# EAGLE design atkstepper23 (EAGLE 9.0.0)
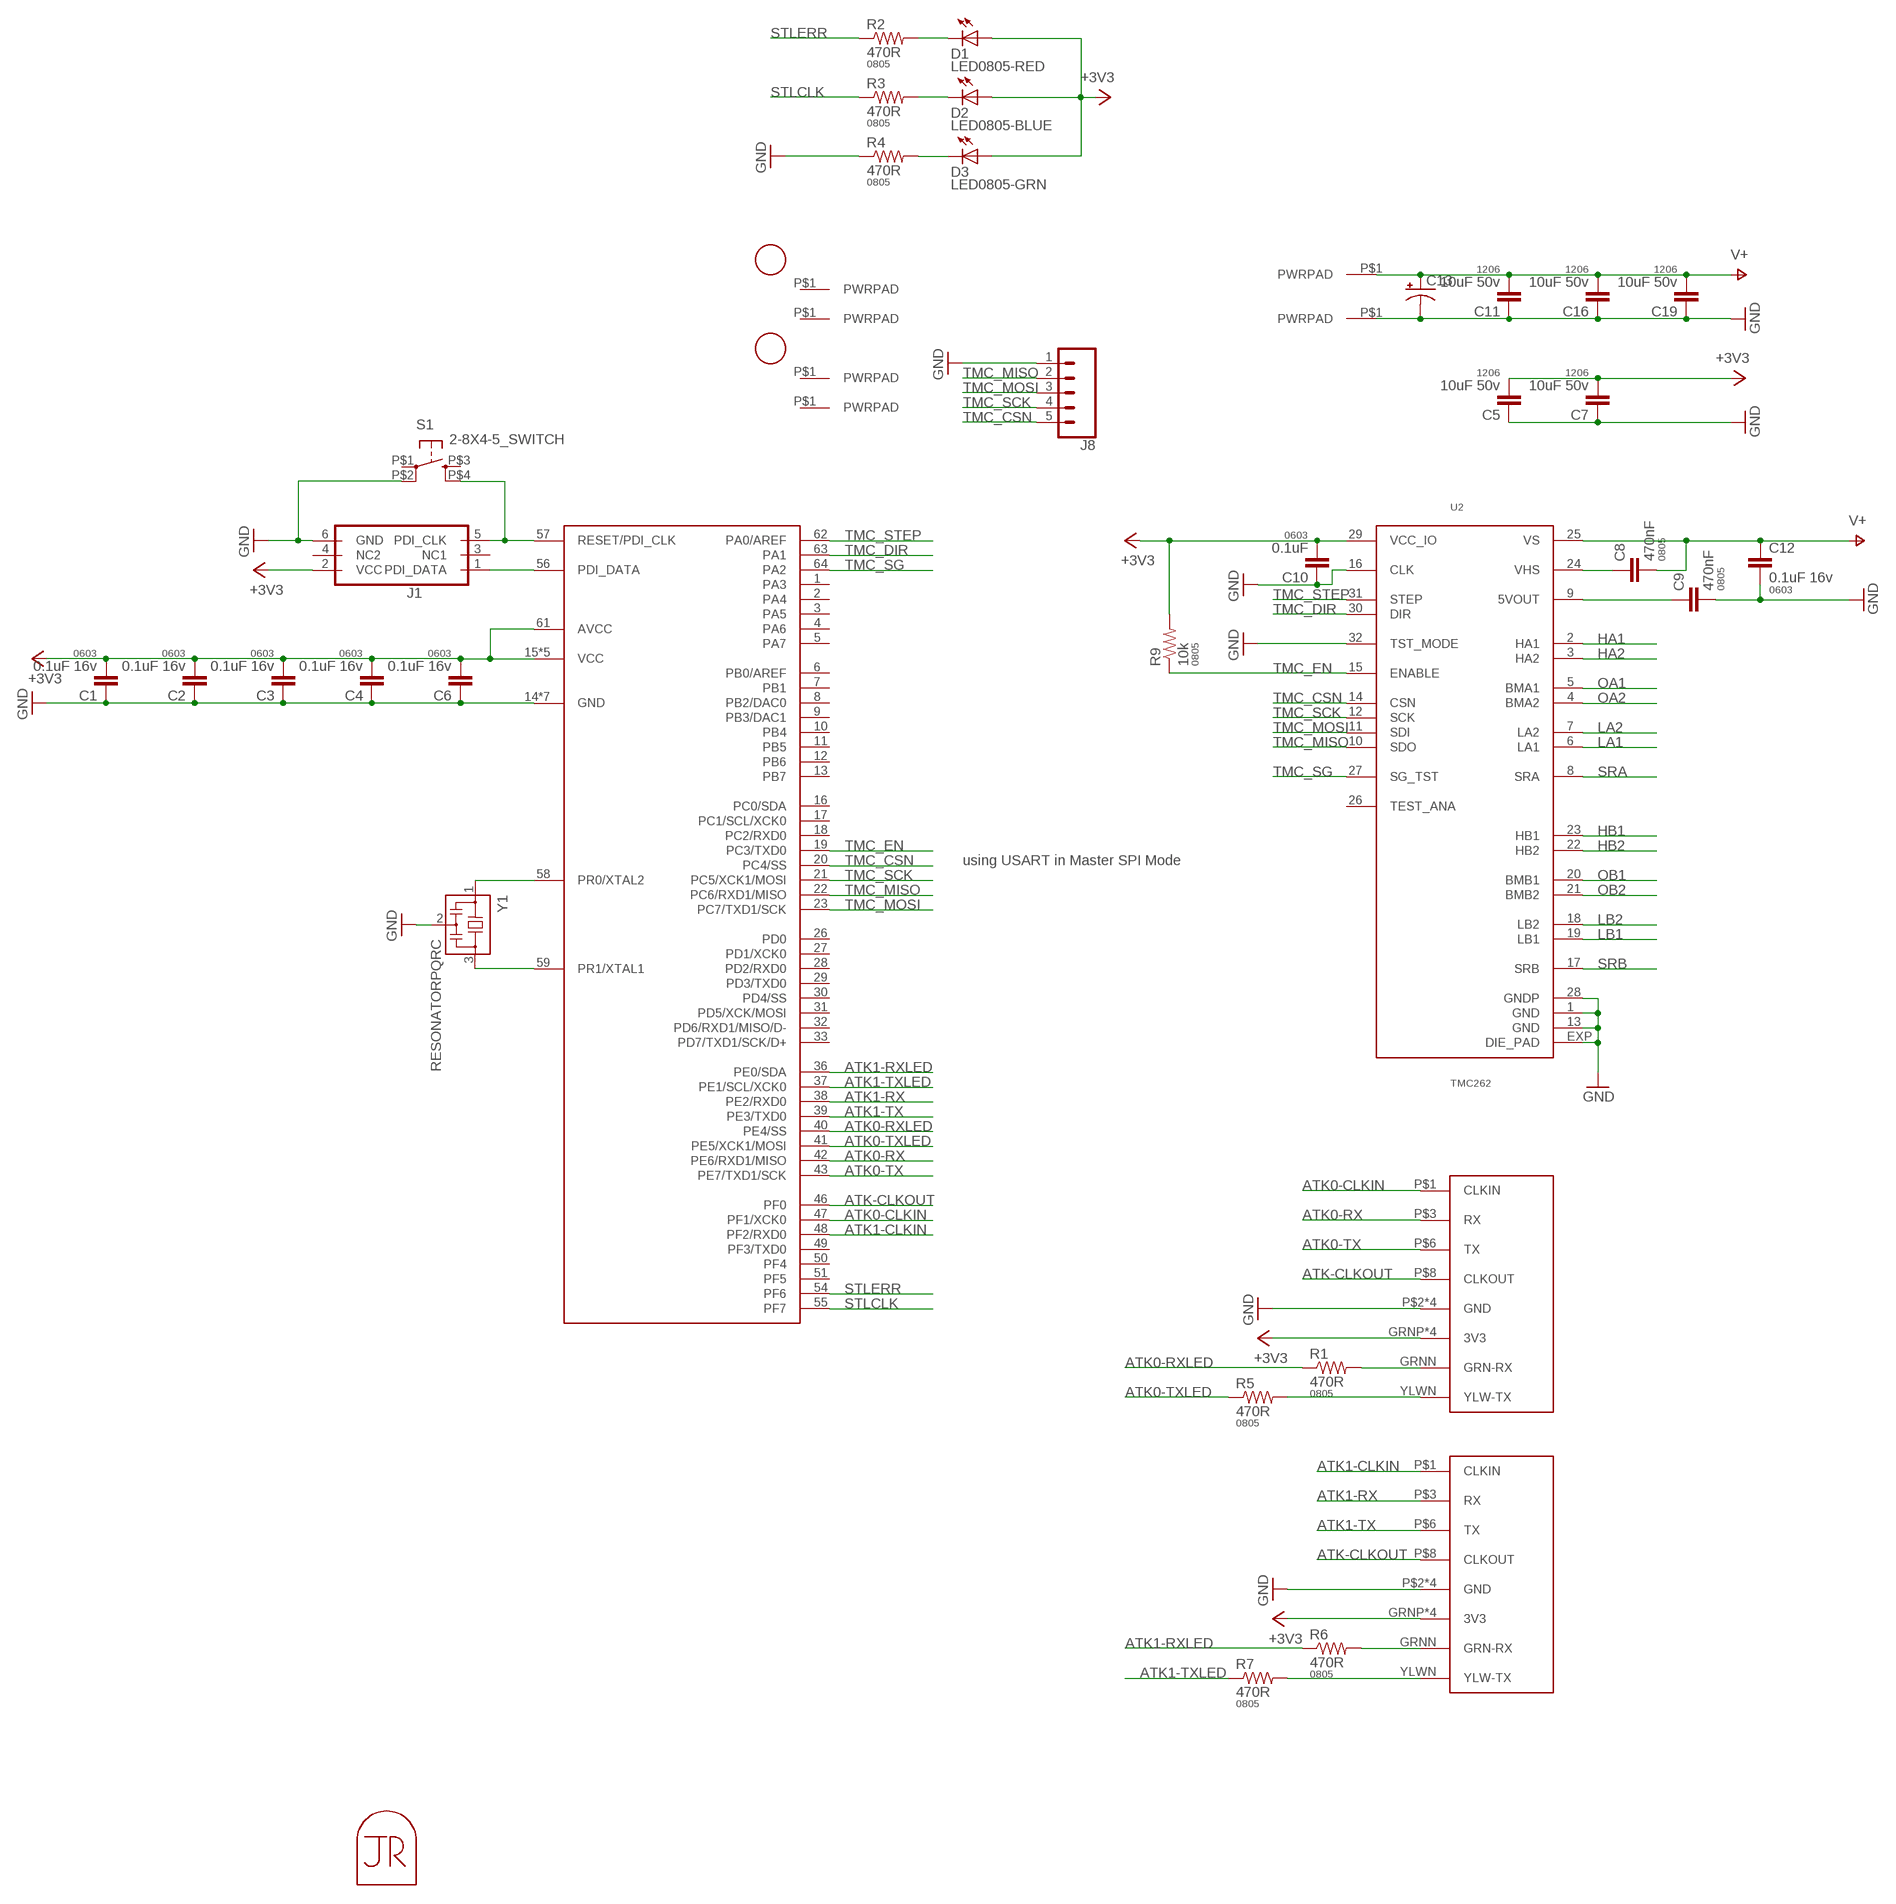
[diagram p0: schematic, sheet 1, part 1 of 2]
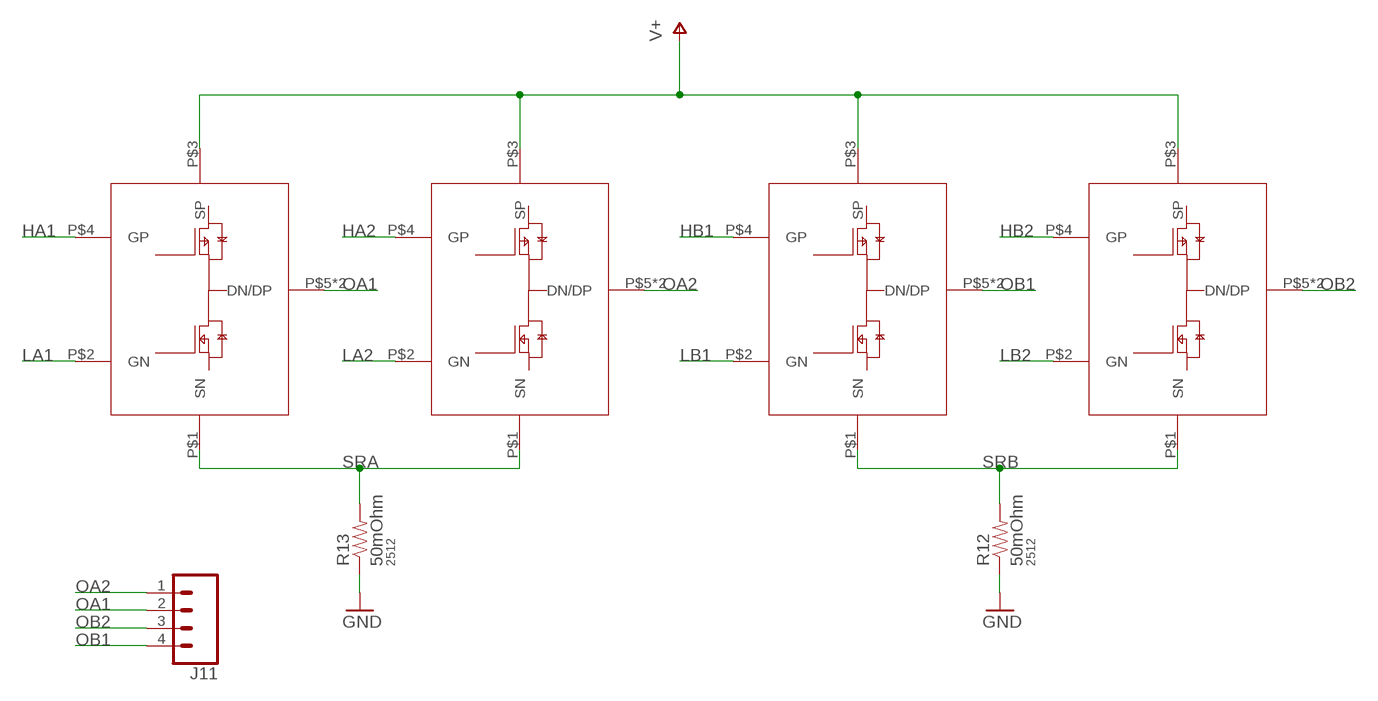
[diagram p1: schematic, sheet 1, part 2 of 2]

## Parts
C1  0.1uF 16v  CAP0603-CAP  [0603-CAP]
C2  0.1uF 16v  CAP0603-CAP  [0603-CAP]
C3  0.1uF 16v  CAP0603-CAP  [0603-CAP]
C4  0.1uF 16v  CAP0603-CAP  [0603-CAP]
C5  10uF 50v  CAP1206  [1206]
C6  0.1uF 16v  CAP0603-CAP  [0603-CAP]
C7  10uF 50v  CAP1206  [1206]
C8  470nF  CAP0805  [0805]
C9  470nF  CAP0805  [0805]
C10  0.1uF  CAP0603-CAP  [0603-CAP]
C11  10uF 50v  CAP1206  [1206]
C12  0.1uF 16v  CAP0603-CAP  [0603-CAP]
C13  CAP-POL-6.6X6.6  [6.6X6.6-CAP]
C16  10uF 50v  CAP1206  [1206]
C19  10uF 50v  CAP1206  [1206]
D1  LED0805-RED  LED0805  [LED0805]
D2  LED0805-BLUE  LED0805  [LED0805]
D3  LED0805-GRN  LED0805  [LED0805]
J1  PDIFEMALE_SMD  [PDI_2X3_SMD]
J2  ATK-PHY  [RJ45-LED-RJE7318800XXX]
J3  ATK-PHY  [RJ45-LED-RJE7318800XXX]
J4  PWRPADM3-SKINNY  [PWRPAD_3-25MM-SKINNY]
J6  PWRPADM3-SKINNY  [PWRPAD_3-25MM-SKINNY]
J8  CONN_05NO_SILK  [1X05_NO_SILK]
J9  PWRPAD  [PWRPAD_M3-PEM-MOUNT]
J10  PWRPAD  [PWRPAD_M3-PEM-MOUNT]
J11  CONN_04LONGPADS  [1X04_LONGPADS]
J12  PWRPADM3-SKINNY  [PWRPAD_3-25MM-SKINNY]
J13  PWRPADM3-SKINNY  [PWRPAD_3-25MM-SKINNY]
MP1  JRTOMBSTONE  [JRTOMBSTONE]
Q1  PNPAIR-STL40C30H3LL-FDD8424HSTM  [POWERFLAT-5X6]
Q2  PNPAIR-STL40C30H3LL-FDD8424HSTM  [POWERFLAT-5X6]
Q3  PNPAIR-STL40C30H3LL-FDD8424HSTM  [POWERFLAT-5X6]
Q4  PNPAIR-STL40C30H3LL-FDD8424HSTM  [POWERFLAT-5X6]
R1  470R  RESISTOR0805-RES  [0805]
R2  470R  RESISTOR0805-RES  [0805]
R3  470R  RESISTOR0805-RES  [0805]
R4  470R  RESISTOR0805-RES  [0805]
R5  470R  RESISTOR0805-RES  [0805]
R6  470R  RESISTOR0805-RES  [0805]
R7  470R  RESISTOR0805-RES  [0805]
R9  10k  RESISTOR0805-RES  [0805]
R12  50mOhm  RESISTOR2512  [R2512]
R13  50mOhm  RESISTOR2512  [R2512]
S1  2-8X4-5_SWITCH  [TACT-SWITCH-KMR6]
U1  ATXMEGA_A3UQFN  [QFN-64-9X9MM]
U2  TMC262  [QFN32]
U$1  FIDUCIAL  [FIDUCIAL_1MM]
U$2  FIDUCIAL  [FIDUCIAL_1MM]
Y1  RESONATORPQRC  [RES_PRQC]

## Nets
+3V3: C1.2 C2.2 C3.2 C4.2 C5.2 C6.2 C7.2 C10.2 D1.1(A) D2.1(A) D3.1(A) J1.2(VCC) J2.GRNP(3V3) J2.P$4(3V3) J2.P$5(3V3) J2.YLWP(3V3) J3.GRNP(3V3) J3.P$4(3V3) J3.P$5(3V3) J3.YLWP(3V3) R9.2 U1.15(VCC) U1.25(VCC) U1.35(VCC) U1.45(VCC) U1.53(VCC) U1.61(AVCC) U2.29(VCC_IO)
ATK0-CLKIN: J2.P$1(CLKIN) U1.47(PF1/XCK0)
ATK0-RX: J2.P$3(RX) U1.42(PE6/RXD1/MISO)
ATK0-RXLED: R1.1 U1.40(PE4/SS)
ATK0-TX: J2.P$6(TX) U1.43(PE7/TXD1/SCK)
ATK0-TXLED: R5.1 U1.41(PE5/XCK1/MOSI)
ATK1-CLKIN: J3.P$1(CLKIN) U1.48(PF2/RXD0)
ATK1-RX: J3.P$3(RX) U1.38(PE2/RXD0)
ATK1-RXLED: R6.1 U1.36(PE0/SDA)
ATK1-TX: J3.P$6(TX) U1.39(PE3/TXD0)
ATK1-TXLED: R7.1 U1.37(PE1/SCL/XCK0)
ATK-CLKOUT: J2.P$8(CLKOUT) J3.P$8(CLKOUT) U1.46(PF0)
GND: C1.1 C2.1 C3.1 C4.1 C5.1 C6.1 C7.1 C9.2 C10.1 C11.1 C12.2 C13.- C16.1 C19.1 J1.6(GND) J2.P$2(GND) J2.P$7(GND) J2.SHDL1(GND) J2.SHDL2(GND) J3.P$2(GND) J3.P$7(GND) J3.SHDL1(GND) J3.SHDL2(GND) J8.1 J10.P$1(PWRPAD) R4.1 R12.1 R13.1 S1.P$2(P1) U1.14(GND) U1.24(GND) U1.34(GND) U1.44(GND) U1.52(GND) U1.60(GND) U1.P$1(GND) U2.1(GND) U2.13(GND) U2.16(CLK) U2.28(GNDP) U2.32(TST_MODE) U2.EXP(DIE_PAD) Y1.2
HA1: Q1.P$4(GP) U2.2(HA1)
HA2: Q2.P$4(GP) U2.3(HA2)
HB1: Q3.P$4(GP) U2.23(HB1)
HB2: Q4.P$4(GP) U2.22(HB2)
LA1: Q1.P$2(GN) U2.6(LA1)
LA2: Q2.P$2(GN) U2.7(LA2)
LB1: Q3.P$2(GN) U2.19(LB1)
LB2: Q4.P$2(GN) U2.18(LB2)
N$1: D3.2(C) R4.2
N$2: C8.1 U2.24(VHS)
N$3: C9.1 U2.9(5VOUT)
N$4: J1.5(PDI_CLK) S1.P$4(S1) U1.57(RESET/PDI_CLK)
N$5: D2.2(C) R3.2
N$6: D1.2(C) R2.2
N$7: U1.58(PR0/XTAL2) Y1.1
N$8: U1.59(PR1/XTAL1) Y1.3
N$10: J1.1(PDI_DATA) U1.56(PDI_DATA)
N$11: J3.GRNN(GRN-RX) R6.2
N$12: J3.YLWN(YLW-TX) R7.2
N$17: J2.GRNN(GRN-RX) R1.2
N$18: J2.YLWN(YLW-TX) R5.2
OA1: J11.2 Q1.P$5(DN/DP) Q1.P$8(DN/DP) U2.5(BMA1)
OA2: J11.1 Q2.P$5(DN/DP) Q2.P$8(DN/DP) U2.4(BMA2)
OB1: J11.4 Q3.P$5(DN/DP) Q3.P$8(DN/DP) U2.20(BMB1)
OB2: J11.3 Q4.P$5(DN/DP) Q4.P$8(DN/DP) U2.21(BMB2)
SRA: Q1.P$1(SN) Q2.P$1(SN) R13.2 U2.8(SRA)
SRB: Q3.P$1(SN) Q4.P$1(SN) R12.2 U2.17(SRB)
STLCLK: R3.1 U1.55(PF7)
STLERR: R2.1 U1.54(PF6)
TMC_CSN: J8.5 U1.20(PC4/SS) U2.14(CSN)
TMC_DIR: U1.63(PA1) U2.30(DIR)
TMC_EN: R9.1 U1.19(PC3/TXD0) U2.15(ENABLE)
TMC_MISO: J8.2 U1.22(PC6/RXD1/MISO) U2.10(SDO)
TMC_MOSI: J8.3 U1.23(PC7/TXD1/SCK) U2.11(SDI)
TMC_SCK: J8.4 U1.21(PC5/XCK1/MOSI) U2.12(SCK)
TMC_SG: U1.64(PA2) U2.27(SG_TST)
TMC_STEP: U1.62(PA0/AREF) U2.31(STEP)
V+: C8.2 C11.2 C12.1 C13.+ C16.2 C19.2 J9.P$1(PWRPAD) Q1.P$3(SP) Q2.P$3(SP) Q3.P$3(SP) Q4.P$3(SP) U2.25(VS)
Unconnected: J1.3(NC1) J1.4(NC2) J4.P$1(PWRPAD) J6.P$1(PWRPAD) J12.P$1(PWRPAD) J13.P$1(PWRPAD) S1.P$1(P) S1.P$3(S) U1.1(PA3) U1.2(PA4) U1.3(PA5) U1.4(PA6) U1.5(PA7) U1.6(PB0/AREF) U1.7(PB1) U1.8(PB2/DAC0) U1.9(PB3/DAC1) U1.10(PB4) U1.11(PB5) U1.12(PB6) U1.13(PB7) U1.16(PC0/SDA) U1.17(PC1/SCL/XCK0) U1.18(PC2/RXD0) U1.26(PD0) U1.27(PD1/XCK0) U1.28(PD2/RXD0) U1.29(PD3/TXD0) U1.30(PD4/SS) U1.31(PD5/XCK/MOSI) U1.32(PD6/RXD1/MISO/D-) U1.33(PD7/TXD1/SCK/D+) U1.49(PF3/TXD0) U1.50(PF4) U1.51(PF5) U2.26(TEST_ANA)

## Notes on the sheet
- using USART in Master SPI Mode

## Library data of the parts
C1-C4 C6 C10 C12 = borkedlabs-passives:CAP: Capacitor; PACKAGE: 0603
C5 C7 C11 C16 C19 = borkedlabs-passives:CAP: Capacitor; PACKAGE: 1206
C8 C9 = borkedlabs-passives:CAP: Capacitor; PACKAGE: 0805
C13 = borkedlabs-passives:CAP-POL
D1-D3 = lights:LED: LED
J1 = microcontrollers:PDI: Multi connection point. Often used as Generic Header-pin footprint for 0.1 inch spaced/style header connections You can populate with any combo of single row headers, but if you'd like an exact match, check these: Header - 2x3 (Male, 0.1") (PRT-12807) Header - 2x3 (Female, 0.1") (PRT-13010) 2x3 Pin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; PROD_ID: CONN-11290
J2 J3 = connector:ATK-PHY
J4 J6 J9 J10 J12 J13 = power:PWRPAD
J8 = SparkFun-Connectors:CONN_05: Multi connection point. Often used as Generic Header-pin footprint for 0.1 inch spaced/style header connections On any of the 0.1 inch spaced packages, you can populate with these: Break Away Headers - Straight (PRT-00116) Break Away Male Headers - Right Angle (PRT-00553) Female Headers (PRT-00115)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
J11 = SparkFun-Connectors:CONN_04: Multi connection point. Often used as Generic Header-pin footprint for 0.1 inch spaced/style header connections On any of the 0.1 inch spaced packages, you can populate with these: Break Away Headers - Straight (PRT-00116) Break Away Male Headers - Right Angle (PRT-00553) Female Headers (PRT-00115)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; PROD_ID: CONN-09696
MP1 = connector:JRTOMBSTONE
Q1-Q4 = power:PNPAIR-STL40C30H3LL-FDD8424H
R1-R7 R9 = borkedlabs-passives:RESISTOR: Resistor; PACKAGE: 0805
R12 R13 = borkedlabs-passives:RESISTOR: Resistor; PACKAGE: 2512
S1 = fab:2-8X4-5_SWITCH
U1 = microcontrollers:ATXMEGA_A3U
U2 = power:TMC262
U$1 U$2 = connector:FIDUCIAL: For use by pick and place machines to calibrate the vision/machine, 1mm
Y1 = passives:RESONATOR

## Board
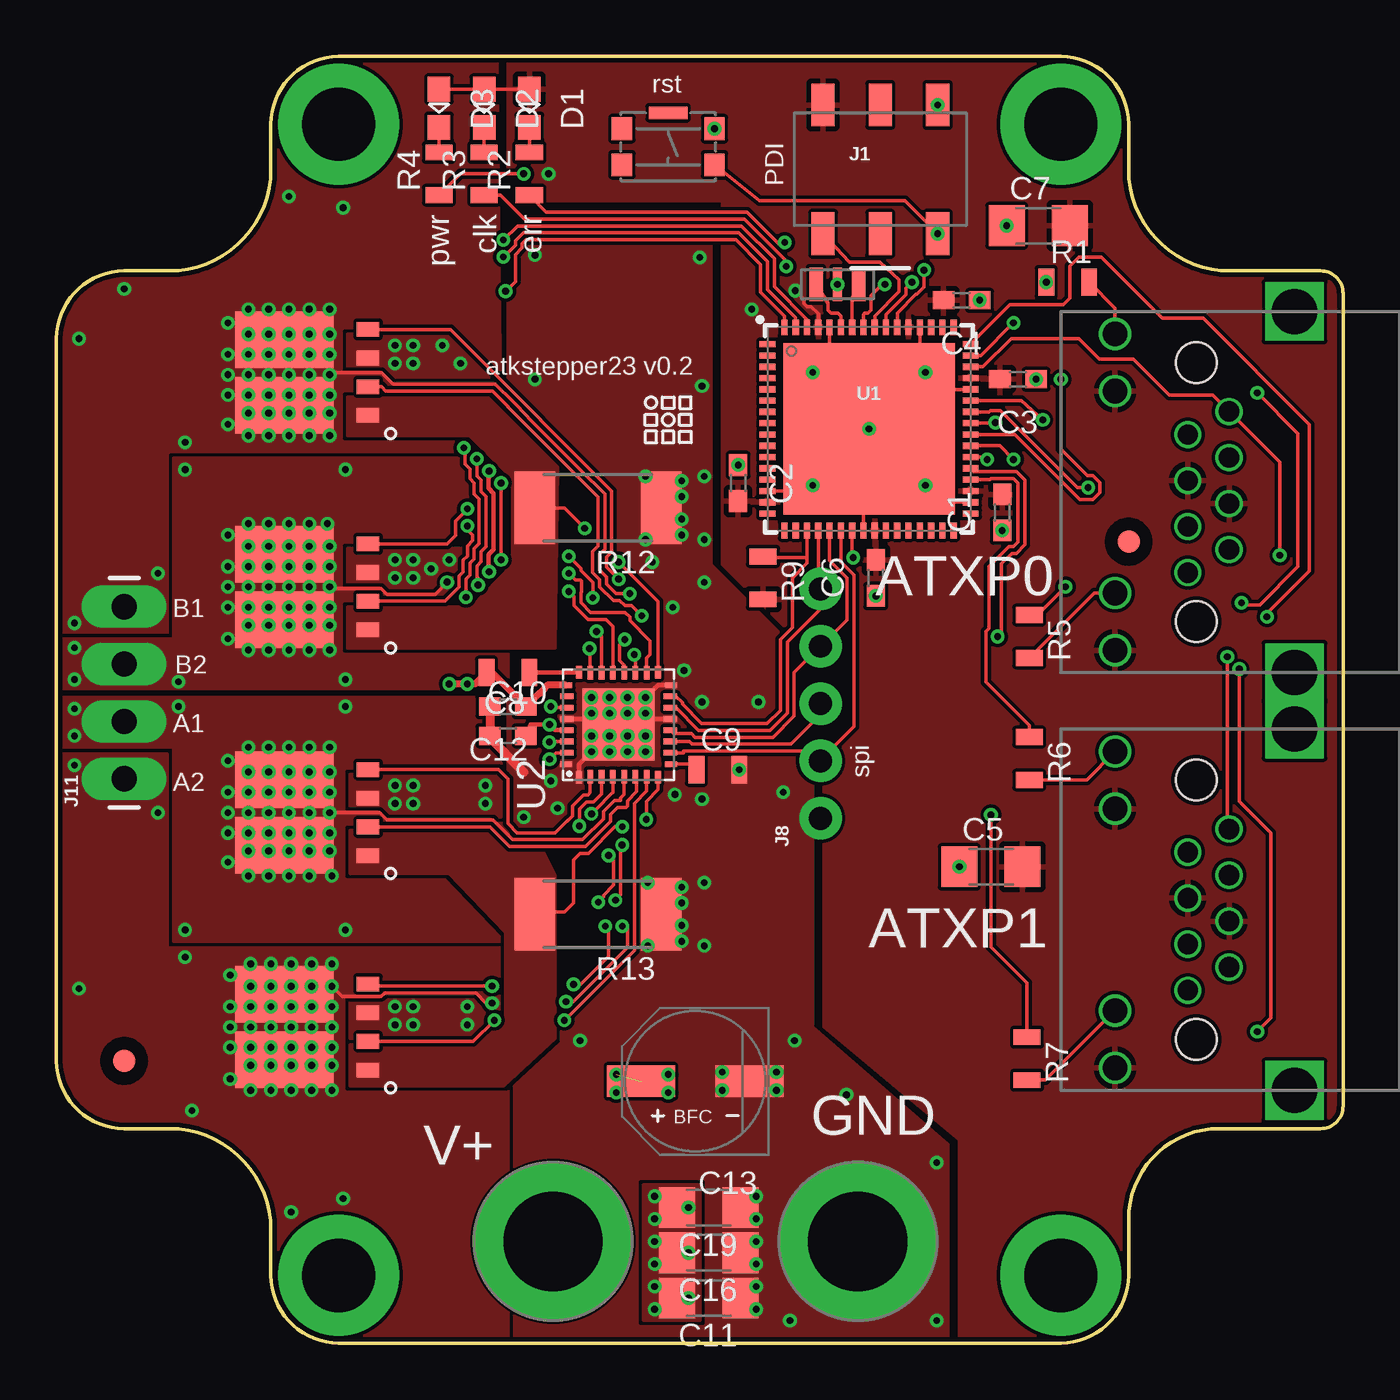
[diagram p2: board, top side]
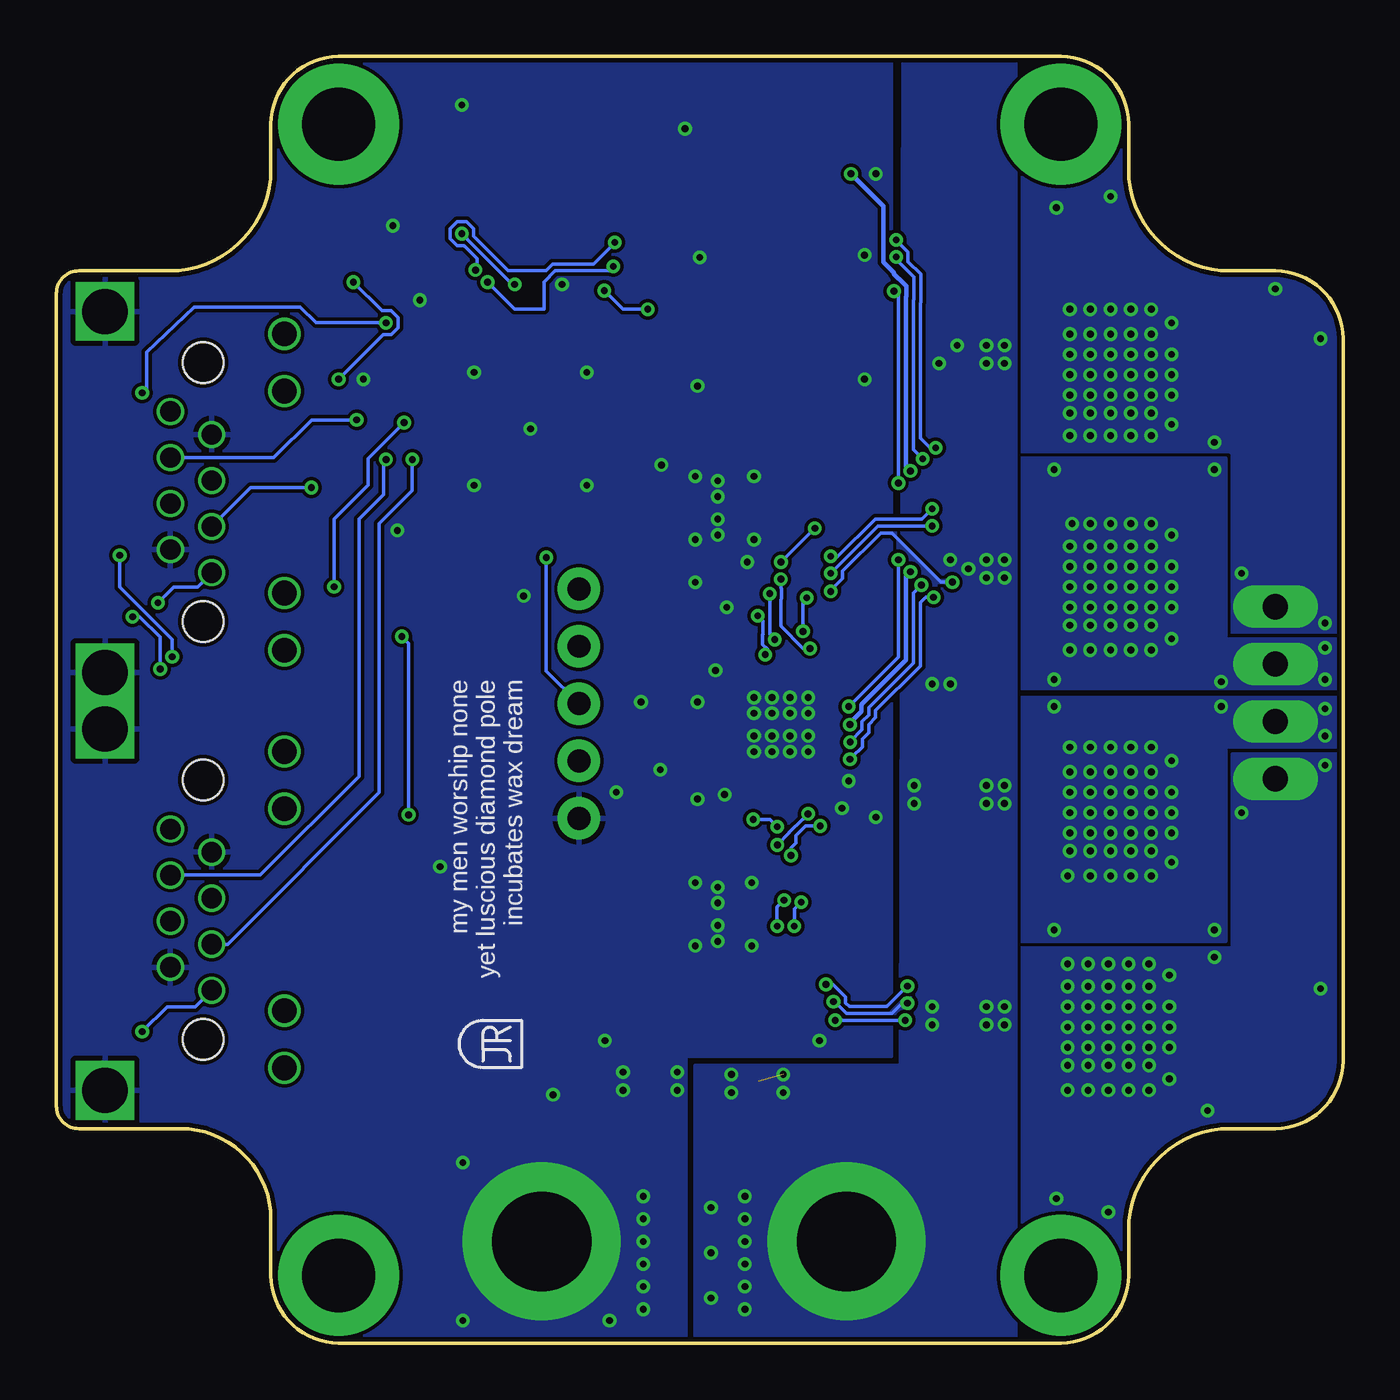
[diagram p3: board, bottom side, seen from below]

Size 57 x 57 mm. Coordinates in mm from the lower left corner, seen from the top.
Outline: 44.5,0 12.5,0 arc-90 9.5,3 9.5,5 arc90 5,9.5 3,9.5 arc-90 0,12.5 0,44.5 arc-90 3,47.5 5,47.5 arc90 9.5,52 9.5,54 arc-90 12.5,57 44.5,57 arc-90 47.5,54 47.5,52 arc90 52,47.5 56,47.5 arc-90 57,46.5 57,10.5 arc-90 56,9.5 51.5,9.5 arc90 47.5,5.5 47.5,3 arc-90 44.5,0
Copper layers (1*16): Top 0.035mm / dielectric 1.5mm / Bottom 0.035mm
Design rules "default *": minimum track width 6mil, minimum drill 0.3mm, track to track 6mil, track to pad 6mil, pad to pad 6mil, via to via 6mil, smd to smd 6mil, copper to edge 8mil, drill to drill 8mil, minimum pad ring 6mil, minimum via ring 6mil, stop-mask expansion 4mil, vias tented up to drill 27mil, thermal gap 9mil

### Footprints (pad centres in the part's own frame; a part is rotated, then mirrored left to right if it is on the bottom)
0603-CAP = smd 0.96 x 0.8: 1 -0.8,0; 2 0.8,0
1206 = smd 1.6 x 1.8: 1 -1.4,0; 2 1.4,0
0805 = smd 0.7 x 1.2: 1 -0.95,0; 2 0.95,0
6.6X6.6-CAP = smd 3 x 1.4: + 2.4,0; - -2.4,0
LED0805 = smd 1.1 x 1: 1 -0.85,0; 2 0.85,0
PDI_2X3_SMD = smd 1.02 x 1.9: 1 -2.54,-2.85; 2 -2.54,2.85; 3 0,-2.85; 4 0,2.85; 5 2.54,-2.85; 6 2.54,2.85
RJ45-LED-RJE7318800XXX = drill 1.1: GRNN 7.01,3.6; GRNP 4.47,3.6; YLWN -4.47,3.6; YLWP -7.01,3.6 | drill 0.9: P$1 -3.57,0.38; P$2 -2.55,-1.45; P$3 -1.53,0.38; P$4 -0.51,-1.45; P$5 0.51,0.38; P$6 1.53,-1.45; P$7 2.55,0.38; P$8 3.57,-1.45 | drill 2 square: SHDL1 -8,-4.35; SHDL2 8,-4.35 | hole 1.8: -5.74,0; 5.74,0
PWRPAD_3-25MM-SKINNY = drill 3.25 pad 5.35: P$1 0,0
1X05_NO_SILK = drill 1.016 pad 1.88: 1 0,0; 2 2.54,0; 3 5.08,0; 4 7.62,0; 5 10.16,0
PWRPAD_M3-PEM-MOUNT = drill 4.4 pad 7: P$1 0,0
1X04_LONGPADS = drill 1.118 pad 1.88 long: 1 0,0; 2 2.54,0; 3 5.08,0; 4 7.62,0
POWERFLAT-5X6 = smd 0.65 x 1: P$1 -1.905,-2.8; P$2 -0.635,-2.8; P$3 0.635,-2.8; P$4 1.905,-2.8 | smd 2.5 x 4.35: P$5 1.45,0.9; P$8 -1.45,0.9
R2512 = smd 1.8 x 3.2: 1 -2.8,0; 2 2.8,0
TACT-SWITCH-KMR6 = smd 0.9 x 1: P$1 -2.05,0.8; P$2 2.05,0.8; P$3 -2.05,-0.8; P$4 2.05,-0.8 | smd 1.7 x 0.55: P$5 0,1.5
QFN-64-9X9MM = smd 0.7 x 0.275: 1 -4.5,3.75; 2 -4.5,3.25; 3 -4.5,2.75; 4 -4.5,2.25; 5 -4.5,1.75; 6 -4.5,1.25; 7 -4.5,0.75; 8 -4.5,0.25; 9 -4.5,-0.25; 10 -4.5,-0.75; 11 -4.5,-1.25; 12 -4.5,-1.75; 13 -4.5,-2.25; 14 -4.5,-2.75; 15 -4.5,-3.25; 16 -4.5,-3.75; 33 4.5,-3.75; 34 4.5,-3.25; 35 4.5,-2.75; 36 4.5,-2.25; 37 4.5,-1.75; 38 4.5,-1.25; 39 4.5,-0.75; 40 4.5,-0.25; 41 4.5,0.25; 42 4.5,0.75; 43 4.5,1.25; 44 4.5,1.75; 45 4.5,2.25; 46 4.5,2.75; 47 4.5,3.25; 48 4.5,3.75 | smd 0.275 x 0.7: 17 -3.75,-4.5; 18 -3.25,-4.5; 19 -2.75,-4.5; 20 -2.25,-4.5; 21 -1.75,-4.5; 22 -1.25,-4.5; 23 -0.75,-4.5; 24 -0.25,-4.5; 25 0.25,-4.5; 26 0.75,-4.5; 27 1.25,-4.5; 28 1.75,-4.5; 29 2.25,-4.5; 30 2.75,-4.5; 31 3.25,-4.5; 32 3.75,-4.5; 49 3.75,4.5; 50 3.25,4.5; 51 2.75,4.5; 52 2.25,4.5; 53 1.75,4.5; 54 1.25,4.5; 55 0.75,4.5; 56 0.25,4.5; 57 -0.25,4.5; 58 -0.75,4.5; 59 -1.25,4.5; 60 -1.75,4.5; 61 -2.25,4.5; 62 -2.75,4.5; 63 -3.25,4.5; 64 -3.75,4.5 | smd 7.6 x 7.6: P$1 0,0
QFN32 = smd 0.55 x 0.25: 1 -2.325,1.75; 8 -2.325,-1.75; 17 2.325,-1.75; 24 2.325,1.75 | smd 0.6 x 0.25: 2 -2.3,1.25; 3 -2.3,0.75; 4 -2.3,0.25; 5 -2.3,-0.25; 6 -2.3,-0.75; 7 -2.3,-1.25; 18 2.3,-1.25; 19 2.3,-0.75; 20 2.3,-0.25; 21 2.3,0.25; 22 2.3,0.75; 23 2.3,1.25 | smd 0.25 x 0.55: 9 -1.75,-2.325; 16 1.75,-2.325; 25 1.75,2.325; 32 -1.75,2.325 | smd 0.25 x 0.6: 10 -1.25,-2.3; 11 -0.75,-2.3; 12 -0.25,-2.3; 13 0.25,-2.3; 14 0.75,-2.3; 15 1.25,-2.3; 26 1.25,2.3; 27 0.75,2.3; 28 0.25,2.3; 29 -0.25,2.3; 30 -0.75,2.3; 31 -1.25,2.3 | smd 3.2 x 3.2: EXP 0,0
FIDUCIAL_1MM = smd 1 x 1: 1 0,0
RES_PRQC = smd 0.6 x 1.5: 1 -0.95,0; 3 0.95,0 | smd 0.4 x 1.5: 2 0,0

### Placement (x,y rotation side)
C1  41.9,36.8 90 top
C2  30.2,38.1 270 top
C3  42.6,42.7 180 top
C4  40.1,46.2 180 top
C5  41.4,21.1 0 top
C6  36.3,33.9 90 top
C7  43.5,49.5 0 top
C8  20,29.7 180 top
C9  29.3,25.4 0 top
C10  20,26.9 0 top
C11  28.9,2 180 top
C12  20,28.2 180 top
C13  28.3,11.6 180 top
C16  28.9,4 180 top
C19  28.9,6 180 top
D1  20.95,54.7 270 top
D2  18.95,54.7 270 top
D3  16.95,54.7 270 top
J1  36.5,52 0 top
J2  50.5,37.7 90 top
J3  50.5,19.2 90 top
J4  12.5,3 180 top
J6  44.5,3 180 top
J8  33.85,23.25 90 top
J9  22,4.5 180 top
J10  35.5,4.5 180 top
J11  3,25 90 top
J12  12.5,54 180 top
J13  44.5,54 180 top
MP1  37.4,13.3 90 bottom
Q1  11,23.5 90 top
Q2  11,14 90 top
Q3  11,43 90 top
Q4  11,33.5 90 top
R1  44.8,47 0 top
R2  20.95,51.8 90 top
R3  18.95,51.8 90 top
R4  16.95,51.8 90 top
R5  43.1,31.3 270 top
R6  43.1,25.9 270 top
R7  43,12.6 270 top
R9  31.3,33.9 270 top
R12  24,37 180 top
R13  24,19 180 top
S1  27.1,53 0 top
U1  36,40.5 0 top
U2  24.9,27.4 90 top
U$1  3,12.5 0 top
U$2  47.5,35.5 0 top
U$5  [CBA-SILK-LOGO]  27.1,40.9 0 top
Y1  34.6,46.9 180 top

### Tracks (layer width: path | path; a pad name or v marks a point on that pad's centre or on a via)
+3V3  (via drill 0.3)
  Top 0.152: D1.1 D2.1 D3.1 | U1.61 33.75,45.6 33.43,45.92 33.26,45.92 33.12,46.05 33.12,46.23 v32.73,46.62
  Top 0.203: U2.29 22.09,27.15 v21.84,27.4 21,27.4 C10.2 | v19.16,34.16 19.16,34.45 19.14,34.47 19.14,34.93 19.37,35.16 19.37,37.64 19.14,37.87 19.14,38.33 19.16,38.35 v19.16,38.63
  Bottom 0.152: v32.73,46.62 31.9,45.8 v30.8,45.8
  Bottom 0.203: v21.84,27.4 21.84,27.47 21.34,27.97 21.34,28.29 19.37,30.26 19.37,33.96 v19.16,34.16 | v19.16,38.63 19.37,38.84 19.37,46.34 19.34,46.37 19.34,46.83 19.67,47.16 19.7,47.16 19.9,47.36 19.9,47.43 20.36,47.88 20.36,50.36 v21.8,51.8
  pour Top (rank 2): 20,58 20,50.6 29.5,50.6 29.5,34.5 34,30 34,14 40,9 40,-1 57.8,-0.8 57.8,58
ATK0-CLKIN  (via drill 0.3)
  Top 0.152: U1.47 40.95,43.75 v42.4,45.2 | v53.2,42.1 55,40.3 55,34.4 53.3,32.7 52.6,32.7 v52.5,32.8
  Bottom 0.152: v53.2,42.1 53,42.3 53,43.9 50.9,45.9 46.2,45.9 45.5,45.2 v42.4,45.2 | v52.5,32.8 51.8,33.5 50.75,33.5 J2.P$1
ATK0-RX  (via drill 0.3)
  Top 0.152: U1.42 41.32,41.25 41.38,41.31 41.82,41.31 45.23,37.9 v45.7,37.9
  Bottom 0.152: v45.7,37.9 48.39,37.9 J2.P$3
ATK0-RXLED  (via drill 0.3)
  Top 0.152: U1.40 42.45,40.25 45.33,37.37 45.92,37.37 46.23,37.68 46.23,38.12 45.92,38.43 45.68,38.43 44.5,39.61 v44.5,42.7
  Bottom 0.152: R1.1 42.58,45.73 42.18,45.73 41.87,45.42 41.87,44.98 42.18,44.67 42.53,44.67 v44.5,42.7
  other vias: 43.85,47
ATK0-TX  (via drill 0.3)
  Top 0.152: U1.43 42.75,41.75 v43.7,40.9
  Bottom 0.152: J2.P$6 47.37,39.23 45.7,40.9 v43.7,40.9
ATK0-TXLED  (via drill 0.3)
  Top 0.152: U1.41 41.57,40.75 v41.6,40.78 | v44.7,33.5 43.45,32.25 R5.1
  Bottom 0.152: v41.6,40.78 43.2,39.18 43.2,38 44.7,36.5 v44.7,33.5
ATK1-CLKIN  (via drill 0.3)
  Top 0.152: v53.2,13.8 53.8,14.4 53.8,22.6 52.4,24 v52.4,29.86 | U1.48 42.25,46 44.6,46 44.9,46.3 44.9,47.7 45.3,48.1 46.3,48.1 49,45.4 50.8,45.4 55.5,40.7 55.5,34.2 53.62,32.33 v53.62,32.17
  Bottom 0.152: v53.2,13.8 52.1,14.9 50.85,14.9 J3.P$1 | v53.62,32.17 53.31,32.17 52.4,31.27 v52.4,29.86
ATK1-RX  (via drill 0.3)
  Top 0.152: U1.38 41.13,39.25 v41.24,39.14
  Bottom 0.152: v41.24,39.14 41.24,37.76 42.7,36.3 42.7,24.39 49.42,17.67 J3.P$3
ATK1-RXLED
  Top 0.152: U1.36 41.35,38.25 41.41,38.31 42.4,38.31 42.6,38.1 42.6,35.5 42.4,35.29 42.19,35.29 41.3,34.4 41.3,31.65 41.17,31.52 41.17,29.28 43.1,27.35 R6.1
ATK1-TX  (via drill 0.3)
  Top 0.152: U1.39 41.79,39.75 v42.4,39.14
  Bottom 0.152: v42.4,39.14 42.5,39.04 42.5,37.6 43.6,36.5 43.6,25.1 47.97,20.73 J3.P$6
ATK1-TXLED  (via drill 0.3)
  Top 0.152: U1.37 40.63,38.62 40.95,38.62 40.95,38.61 42.52,38.61 42.91,38.23 42.91,35.37 42.52,34.99 42.32,34.99 41.87,34.53 41.87,31.47 v41.7,31.3 | v41.4,23.4 41.4,17.55 43,15.95 R7.1
  Bottom 0.152: v41.7,31.3 41.4,31 v41.4,23.4
ATK-CLKOUT  (via drill 0.3)
  Top 0.152: U1.46 41.05,43.25 42.3,44.5 45.3,44.5 46.2,43.6 47.7,43.6 49.3,42 51.22,42 J2.P$8 54.2,39.02 v54.2,34.9 | v51.87,30.4 51.87,23.19 J3.P$8
  Bottom 0.152: v54.2,34.9 54.2,33.5 51.87,31.17 v51.87,30.4
GND  (via drill 0.3)
  Top 0.152: R4.1 17.9,51.8 v20.7,51.8 | U1.60 34.25,42.25 35.9,40.6 | 35.9,40.6 U1.P$1 36.05,40.55 | U1.52 38.25,42.75 36.05,40.55 | U1.34 39.35,37.25 36.05,40.55 | U1.24 35.75,40.4 | 35.75,40.4 35.75,40.45 35.9,40.6 | U1.14 33.1,37.75 35.75,40.4 | U1.44 39.25,42.25 v38.5,43
  Top 0.203: U2.1 23.15,25.65 v23.7,26.2 | U2.13 26.35,27.65 v26.1,27.9 | U2.16 26.65,29.15 v26.1,28.6 | U2.28 23.45,27.65 v23.7,27.9
  Top 0.406: C12.2 C10.1 19.2,26.8 20.7,25.3
  other vias: 26.1,26.2 24.5,26.2 25.3,26.2 26.1,26.9 23.7,26.9 24.5,26.9 25.3,26.9 24.5,27.9 25.3,27.9 23.7,28.6 24.5,28.6 25.3,28.6 27.7,17.8 27.7,18.5 27.7,19.5 27.7,20.2 28.7,20.4 28.7,17.6 26.2,17.6 26.2,20.4 27.7,35.8 27.7,36.5 27.7,37.5 27.7,38.2 28.7,38.4 28.7,35.6 26.1,35.6 26.1,38.4 30.25,25.4 27.8,29.8 28.6,28.4 26.4,34.6 21.2,42.7 28.6,42.4 28.5,48.1 21.2,48.2 27.4,24.3 28.6,24.1 31.9,11.2 35,11 31.9,12 39,8 39,1 32.5,1 29.5,11.2 23.2,13.4 20.7,23.3 21.9,24.9 40.9,46.2 41.9,36 30.2,38.9 36.3,33.1 31,1.5 31,2.5 31,3.5 31,4.5 31,5.5 31,6.5 29.5,12 22.2,23.7 27.3,32.6 28.7,33.7 34.6,46.9 29.15,53.8 39.04,54.85 36,40.5 33.5,43 38.5,38 33.5,38 43.4,42.7 42.1,49.5 40,21.1 31.1,28.4 32.2,24.4 32.7,13.4
  pour Bottom: 29.1,-0.5 29.1,12.7 20,12.7 20,59.6 29.5,59.5 59.5,59.5 59,-0.5
  pour Top (no thermals): 25.8,35.3 29,35.3 29,38.7 25.8,38.7
  pour Top (no thermals): 25.8,17.3 29,17.3 29,20.7 25.8,20.7
  pour Top (rank 6, no thermals): 39.5,-1 39.5,8.8 33.5,14 33.5,30 29,34.5 29,50.1 20,50.1 20,-1
HA1
  Top 0.152: U2.2 23.65,24.39 23.54,24.28 23.36,24.28 22.86,23.79 22.86,23.36 22.64,23.13 22.64,23.14 22.1,22.61 20.4,22.61 20,23.01 20,25 19.59,25.41 Q1.P$4
HA2  (via drill 0.3)
  Top 0.152: v22.91,15.89 23.23,15.89 24.47,17.13 24.47,18.31 v24.31,18.47 | v24.01,19.53 24.23,19.76 24.23,19.84 24.69,20.29 24.69,21.37 v24.46,21.6 | v23.17,22.91 23.17,23.66 23.48,23.98 23.8,23.98 24.15,24.32 U2.3 | v19.3,15.81 13.89,15.81 Q2.P$4
  Bottom 0.152: v19.3,15.81 20.2,14.91 21.87,14.91 22.04,15.08 22.04,15.35 22.59,15.89 v22.91,15.89 | v24.31,18.47 24.31,19.23 v24.01,19.53 | v24.46,21.6 24.46,21.94 24.23,22.16 24.23,22.48 23.81,22.91 v23.17,22.91
HB1  (via drill 0.3)
  Top 0.152: v24.91,33.84 24.37,34.38 24.37,34.82 24.6,35.05 | 24.6,35.05 | 24.6,35.05 24.6,37.74 21.45,40.89 21.45,40.92 20.54,41.83 20.44,41.92 20.44,41.93 20.38,41.98 17.46,44.91 Q3.P$4 | U2.23 23.65,30.74 v23.62,30.77
  Bottom 0.152: v24.91,33.84 24.91,33.46 24.87,33.42 24.87,32.98 24.91,32.94 24.91,31.75 23.92,30.77 v23.62,30.77
HB2  (via drill 0.3)
  Top 0.152: v18.2,36.96 v18.2,36.95 17.67,36.42 17.67,35.77 17.3,35.4 Q4.P$4 | v22.7,34.86 v22.7,34.85 23.23,34.32 23.23,34.23 23.76,33.69 v23.76,33.02 | v23.93,31.53 24.15,31.31 U2.22
  Bottom 0.152: v18.2,36.96 18.66,36.51 20.73,36.51 22.42,34.82 22.66,34.82 v22.7,34.86 | v23.93,31.53 23.93,32.85 v23.76,33.02
LA1
  Top 0.152: U2.6 25.7,25.05 25.7,24.43 25.3,24.03 25.3,23.8 25.23,23.73 24.85,23.73 24.54,23.42 24.54,23.1 23.44,22 20.07,22 19.21,22.86 Q1.P$2
LA2  (via drill 0.3)
  Top 0.152: v22.5,14.3 25.6,17.4 25.6,23.9 26.15,24.45 U2.7 | Q2.P$2 18.46,13.37 v19.4,14.3
  Bottom 0.152: v19.4,14.3 v22.5,14.3
LB1  (via drill 0.3)
  Top 0.152: U2.19 25.65,30.45 v25.6,30.5 | v25.93,32.22 25.48,32.67 25.18,32.67 24.95,32.9 24.67,32.9 24.07,33.5 24.07,33.82 23.76,34.13 23.76,35.07 23.99,35.3 23.99,37.48 20.01,41.46 20.01,41.49 19.32,42.18 14.59,42.18 14.4,42.37 Q3.P$2
  Bottom 0.152: v25.6,30.5 25.5,30.6 25.5,30.74 25.71,30.95 25.71,31.39 25.7,31.4 25.7,31.99 v25.93,32.22
LB2  (via drill 0.3)
  Top 0.152: v18.2,36.2 18.2,36.03 18.43,35.8 18.43,35.55 18.2,35.32 18.2,34.87 18.02,34.69 18.02,34.16 17.84,33.97 17.84,33.49 17.21,32.87 Q4.P$2 | U2.18 26.15,30.35 26.3,30.5 26.3,31.1 25.4,32 25.4,32.16 25.2,32.36 23.67,32.36 23.23,32.8 23.23,33.24 23.26,33.27 23.26,33.76 23.23,33.8 23,33.8 v22.7,34.1
  Bottom 0.152: v18.2,36.2 20.6,36.2 v22.7,34.1
N$1
  Top 0.152: D3.2 R4.2
N$2
  Top 0.203: U2.24 23.12,29.7 C8.1
N$3
  Top 0.152: U2.9 28.35,25.65 C9.1
N$4  (via drill 0.3)
  Top 0.152: U1.57 35.75,45.57 35.8,45.62 35.95,45.62 36.08,45.76 36.08,46.4 36.58,46.9 v36.7,46.9 | S1.P$4 31.15,50.6 37.59,50.6 J1.5
  Bottom 0.152: J1.5 38.81,48.92 38.81,48.91 36.8,46.9 v36.7,46.9
  other vias: 39.04,49.15
N$5
  Top 0.152: D2.2 R3.2
N$6
  Top 0.152: D1.2 R2.2
N$7
  Top 0.152: U1.58 35.25,46.3 Y1.1
N$8
  Top 0.152: U1.59 34.75,45.5 34.63,45.62 34.3,45.62 34.17,45.76 34.17,46.08 Y1.3
N$10
  Top 0.152: J1.1 35.13,47.88 36.47,47.88 37.33,47.12 37.33,46.58 36.25,45.5 U1.56
N$11
  Top 0.152: J3.GRNN 45.64,24.95 R6.2
N$12
  Top 0.152: R7.2 43.82,11.65 J3.YLWN
N$17
  Top 0.152: R1.2 46.9,45.85 J2.GRNN
N$18
  Top 0.152: R5.2 45.98,33.23 J2.YLWN
OA1  (via drill 0.3)
  Top 0.152: U2.5 25.15,24.31 24.99,24.15 24.99,24.04 24.72,24.04 24.23,23.55 24.23,23.23 23.31,22.3 20.2,22.3 19.34,23.17 14.64,23.17 14.31,23.5 v12.1,23.5 | 10.51,22.99 Q1.P$5
  other vias: 7.6,21.3 7.6,22.6 7.6,23.5 7.6,24.4 7.6,25.8 12.1,21.8 12.2,20.7 12.1,26.4 12.1,25.3 11.2,21.8 11.2,22.6 11.2,23.5 11.2,24.4 11.2,25.3 10.3,21.8 10.3,20.7 10.3,23.5 10.3,26.4 10.3,25.3 9.4,21.8 9.4,22.6 9.4,23.5 9.4,24.4 9.4,25.3 8.5,21.8 8.5,20.7 8.5,23.5 8.5,26.4 8.5,25.3 12.8,28.2 5.4,28.2 0.8,28.1 0.8,26.9 5.7,18.3 12.8,18.3 8.5,22.6 10.3,22.6 12.1,22.6 11.2,20.7 9.4,20.7 10.3,24.4 12.1,24.4 8.5,24.4 9.4,26.4 11.2,26.4
  pour Top (rank 2, no thermals): -0.3,28.6 20,28.6 20,17.8 5.2,17.8 5.2,26.4 -0.3,26.4
  pour Bottom (rank 2, no thermals): -0.3,28.6 20,28.6 20,17.8 5.2,17.8 5.2,26.4 -0.3,26.4
OA2  (via drill 0.3)
  Top 0.152: v22.57,15.12 22.89,15.12 25.3,17.53 25.3,18.4 25.23,18.47 v25.07,18.47 | v24.76,19.62 24.99,19.85 24.99,22 v25.06,22.07 | U2.4 24.65,24.39 24.6,24.34 | 24.6,24.34 | 23.93,23.67 | 23.93,23.67 v23.7,23.45 | 24.6,24.34 23.93,23.67 | v19.3,15.06 19.04,15.06 18.59,15.51 14.55,15.51 14.39,15.35 12.65,15.35 v12.2,15.8
  Bottom 0.152: v19.3,15.06 19.54,15.06 20,14.61 22,14.61 22.52,15.12 v22.57,15.12 | v25.07,18.47 25.07,19.32 v24.76,19.62 | v23.7,23.45 23.7,23.43 23.91,23.22 23.93,23.22 24.54,22.61 24.54,22.59 v25.06,22.07
  other vias: 7.7,11.7 7.7,13.1 7.7,14 7.7,14.9 7.7,16.3 12.2,12.3 12.2,11.2 12.2,14 5.7,17.1 11.3,12.3 11.3,13.1 11.3,14 11.3,14.9 11.3,15.8 10.4,12.3 10.4,11.2 10.4,14 10.4,16.8 10.4,15.8 9.5,12.3 9.5,13.1 9.5,14 9.5,14.9 9.5,15.8 8.6,12.3 8.6,11.2 8.6,14 8.6,16.8 8.6,15.8 0.8,25.6 4.5,23.5 1,15.7 6,10.3 12.2,16.8 12.7,6.4 10.4,5.8 8.6,13.1 10.4,13.1 12.2,13.1 12.2,14.9 10.4,14.9 8.6,14.9 9.5,16.8 11.3,16.8 11.3,11.2 9.5,11.2
  pour Top (rank 4, no thermals): -0.3,26.1 4.9,26.1 4.9,17.5 20,17.5 20,-1.5 -0.3,-1.5
  pour Bottom (rank 4, no thermals): -0.3,26.1 4.9,26.1 4.9,17.5 20,17.5 20,-1.1 -0.3,-1.1
OB1  (via drill 0.3)
  Top 0.152: 23.2,38.71 21.05,40.85 20.41,41.52 20.41,41.53 20.32,41.61 20.23,41.7 19.44,42.49 14.91,42.49 14.4,43 12.2,43 v12.1,42.9 | 23.2,38.71 23.2,38.7 | 23.2,38.71 24.3,37.61 24.3,35.18 24.06,34.95 24.06,34.25 24.38,33.94 24.38,33.62 24.8,33.2 v25.4,33.2 | U2.20 25.15,30.05 24.95,30.25 24.95,30.94 v25.18,31.17
  Bottom 0.152: v25.4,33.2 25.4,31.39 v25.18,31.17
  other vias: 7.6,40.7 7.6,42 7.6,42.9 7.6,43.8 7.6,45.2 12.1,41.2 12.1,45.8 12.1,44.7 11.2,41.2 11.2,42 11.2,42.9 11.2,43.8 11.2,44.7 10.3,41.2 10.3,40.2 10.3,42.9 10.3,45.8 10.3,44.7 9.4,41.2 9.4,42 9.4,42.9 9.4,43.8 9.4,44.7 8.5,41.2 8.5,40.2 8.5,42.9 8.5,45.8 8.5,44.7 0.8,31.9 4.5,34.1 5.7,39.9 1,44.5 3,46.7 12.1,40.2 12.7,50.3 10.3,50.8 8.5,43.8 10.3,43.8 12.1,43.8 11.2,45.8 9.4,45.8 9.4,40.2 11.2,40.2 8.5,42 10.3,42 12.1,42
  pour Top (rank 3, no thermals): -0.3,31.5 5,31.5 5,39.5 19.7,39.5 19.5,58.3 -0.5,58.3
  pour Bottom (rank 3, no thermals): -0.3,31.5 5,31.5 5,39.5 20,39.5 20,57.7 -0.3,57.7
OB2  (via drill 0.3)
  Top 0.152: v17.3,33.7 v17.31,33.71 16.77,33.17 14.64,33.17 14.39,33.42 12.18,33.42 v12.1,33.5 | v22.7,33.3 22.93,33.07 22.93,32.67 23.54,32.06 24.34,32.06 24.65,31.75 U2.21
  Bottom 0.152: v17.31,33.71 17.81,33.71 20,35.9 20.47,35.9 22.17,34.2 22.17,33.88 22.7,33.35 v22.7,33.3
  other vias: 7.6,31.2 7.6,32.6 7.6,33.5 7.6,34.4 7.6,35.8 12.1,31.8 12.1,30.7 12,36.3 12.1,35.3 11.2,31.8 11.2,32.6 11.2,33.5 11.2,34.4 11.2,35.3 10.3,31.8 10.3,30.7 10.3,33.5 10.3,36.3 10.3,35.3 9.4,31.8 9.4,32.6 9.4,33.5 9.4,34.4 9.4,35.3 8.5,31.8 8.5,30.7 8.5,33.5 8.5,36.3 8.5,35.3 5.7,38.7 0.8,29.4 0.8,30.8 5.4,29.3 12.8,29.4 12.8,38.7 8.5,34.4 10.3,34.4 12.1,34.4 8.5,32.6 10.3,32.6 12.1,32.6 9.4,30.7 11.2,30.7 9.4,36.3 11.2,36.3
  pour Top (rank 2, no thermals): -0.3,29 20,29 20,39.2 5.2,39.2 5.2,31.2 -0.3,31.2
  pour Bottom (rank 2, no thermals): -0.3,29 20,29 20,39.2 5.2,39.2 5.2,31.2 -0.3,31.2
SRA  (via drill 0.3)
  Top 0.152: R13.2 21.3,19.1 22.5,19.1 22.9,19.5 22.9,21.4 23.2,21.7 23.56,21.7 24.75,22.88 v25.07,22.88 | v26.13,23.2 26.13,24 26.65,24.52 U2.8
  Bottom 0.152: v25.07,22.88 25.39,23.2 v26.13,23.2
  pour Top (no thermals): 13,13.2 18.5,13.2 19.9,14.6 19.9,18.2 17.4,20.8 13,20.8 13,22.7 21.1,22.7 22.1,20.7 22.1,13.5 19.8,11.4 13,11.4
SRB  (via drill 0.3)
  Top 0.152: R12.2 22.5,37 v23.4,36.1 | v24.9,34.6 26.65,32.85 U2.17
  Bottom 0.152: v23.4,36.1 v24.9,34.6
  pour Top (no thermals): 12.9,32.6 18.4,32.6 20.2,34.5 20.2,38.3 18.3,40.2 12.9,40.2 12.9,41.9 19.1,41.9 22.2,38.8 22.1,30.8 12.9,30.8
STLCLK  (via drill 0.3)
  Top 0.152: R3.1 19.68,50.85 20.73,49.8 30.47,49.8 32.33,47.94 v32.33,47.7 | v37.9,47 37.64,46.74 37.64,46.45 36.75,45.56 U1.55
  Bottom 0.152: v32.33,47.7 32.53,47.5 34.9,47.5 35.4,47 35.4,45.8 36.7,45.8 v37.9,47
STLERR  (via drill 0.3)
  Top 0.152: R2.1 21.7,50.1 30.6,50.1 32.1,48.6 v32.26,48.76 | v38.44,47.53 38.44,46.78 38.12,46.47 38.09,46.47 37.25,45.63 U1.54
  Bottom 0.152: v32.26,48.76 33.22,47.8 35.03,47.8 35.32,47.52 36.98,47.52 38.51,49.04 38.51,49.37 38.82,49.68 39.26,49.68 39.57,49.37 39.57,48.93 39.26,48.62 38.95,48.62 38.37,48.03 38.37,47.6 v38.44,47.53
TMC_CSN
  Top 0.152: U2.14 27.45,28.15 28.45,27.14 31.61,27.14 32.38,27.91 32.38,31.05 33.85,32.52 J8.5 33.75,33.51 U1.20
TMC_DIR  (via drill 0.3)
  Top 0.152: U2.30 21.86,26.65 v21.84,26.62 | v18.68,33.58 18.68,33.9 18.63,33.95 18.63,34.43 18.81,34.61 18.81,35.07 19.04,35.29 19.04,37.51 18.81,37.73 18.81,38.24 18.63,38.41 v18.63,39.17 | v19.8,48.11 20.33,48.65 20.33,48.83 20.69,49.19 30.22,49.19 31.5,47.91 31.5,46.67 32.75,45.42 U1.63
  Bottom 0.152: v21.84,26.62 21.84,26.66 21.31,27.18 21.31,27.53 21.01,27.83 21.01,28.15 19.04,30.13 19.04,33.22 v18.68,33.58 | v18.63,39.17 19.04,39.58 19.04,46.21 19.01,46.23 19.01,47.22 19.8,48.01 v19.8,48.11
TMC_EN
  Top 0.152: U2.15 27.45,28.65 27.73,28.37 27.73,28.3 28.58,27.45 31.49,27.45 32.07,28.03 32.07,31.18 32.6,31.7 32.6,33.9 33.25,34.55 33.25,34.8 | 33.25,34.8 U1.19 | R9.1 31.35,34.8 33.25,34.8
TMC_MISO
  Top 0.152: U2.10 27.77,26.15 27.77,26.23 33.41,26.23 33.82,25.82 | 33.82,25.82 J8.2 | U1.22 34.75,34.59 35.32,34.02 35.32,27.32 33.82,25.82
TMC_MOSI  (via drill 0.3)
  Top 0.152: U2.11 28.05,26.65 28.17,26.53 32.53,26.53 33.85,27.85 J8.3 | U1.23 35.25,34.85 v35.3,34.8
  Bottom 0.152: v35.3,34.8 35.3,29.78 J8.3
TMC_SCK
  Top 0.152: U2.12 27.35,27 28.13,27 28.29,26.84 31.74,26.84 32.68,27.78 32.68,29.7 J8.4 35.02,32.04 35.02,33.89 34.25,34.66 U1.21
TMC_SG  (via drill 0.3)
  Top 0.152: U2.27 21.95,28.15 v21.9,28.2 | v19.7,34.7 v19.7,38.1 | v19.9,46.6 20.33,47.03 20.33,48.21 20.64,48.52 20.64,48.7 20.81,48.88 30.09,48.88 31.19,47.78 31.19,46.55 32.25,45.49 U1.64
  Bottom 0.152: v21.9,28.2 19.7,30.4 v19.7,34.7 | v19.7,38.1 19.7,46.4 v19.9,46.6
TMC_STEP  (via drill 0.3)
  Top 0.152: v18.14,33.04 18.14,33.84 18.33,34.03 18.33,34.56 18.51,34.74 18.51,35.19 18.73,35.42 18.73,37.38 18.51,37.61 18.51,38.11 18.33,38.29 18.33,38.72 18.1,38.95 18.1,39.6 v18.04,39.66 | v19.8,48.87 20.42,49.49 30.35,49.49 31.8,48.04 31.8,46.8 33.25,45.35 U1.62 | U2.31 22.13,26.15 v21.84,25.87
  Bottom 0.152: v21.84,25.87 21.62,26.09 21.61,26.09 21.41,26.3 21.4,26.3 21.3,26.4 21.3,26.76 21.01,27.05 21.01,27.41 20.71,27.71 20.71,28.03 18.73,30 18.73,32.8 18.49,33.04 v18.14,33.04 | v18.04,39.66 18.29,39.66 18.73,40.1 18.73,46.08 18.71,46.11 18.71,47.35 19.27,47.91 19.27,48.33 v19.8,48.87
V+  (via drill 0.3)  (1 unrouted)
  Top 0.305: U2.25 21.75,29.15 21.61,29 21.61,28.97 21.43,28.8 21.39,28.8 C12.1 19.3,29.7 C8.2 18.55,29.2 v18.2,29.2 v17.4,29.2
  other vias: 15,34.7 15,44.2 15,14.9 15,23.9 15.8,34.7 15,33.9 15,43.4 24.8,11.9 27.1,11.1 27.1,11.9 24.8,11.1 26.5,6.5 26.5,5.5 26.5,4.5 26.5,3.5 26.5,2.5 26.5,1.5 28,2 28,4 28,6 15,14.1 15.8,14.9 15.8,14.1 18.2,14.9 18.2,14.1 15,24.7 15.8,24.7 15.8,23.9 19,23.9 19,24.7 15.8,33.9 17.4,34.7 16.6,34.3 15.8,43.4 15.8,44.2 17.1,44.2 17.9,43.4
  pour Bottom: 14.5,-0.5 28.7,-0.5 28.7,12.3 19.6,12.3 19.5,57.5 14.5,57.5
  pour Top (rank 2, no thermals): 19.1,15.4 13,15.4 13,13.5 18.4,13.5 19.1,14.2
  pour Top (no thermals): 19.7,25.2 13,25.2 13,23.3 19.7,23.3
  pour Top (no thermals): 18.3,35.2 12.9,35.2 12.9,33 18.3,33
  pour Top (no thermals): 17.4,44.7 12.9,44.7 12.9,42.7 19.4,42.7
  pour Top (no thermals): 28.5,1 26,1 26,7 28.5,7

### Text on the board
tPlace: rst | PDI | pwr | clk | err | atkstepper23 v0.2 | ATXP0 | B1 | B2 | A1 | spi | A2 | ATXP1 | GND | V+
bPlace: my men worship none / yet luscious diamond pole / incubates wax dream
